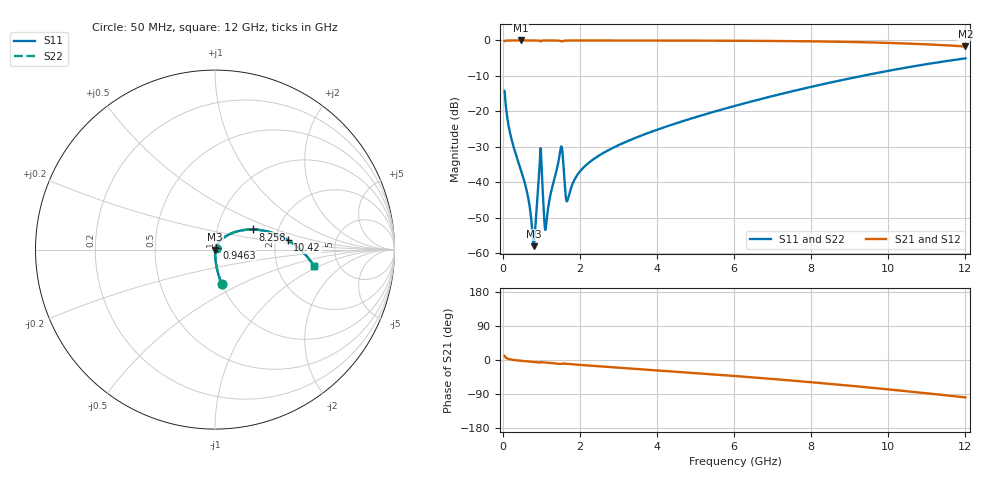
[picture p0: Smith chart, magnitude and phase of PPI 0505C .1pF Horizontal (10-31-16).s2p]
# MHz S MA R 50
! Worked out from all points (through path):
!   1601 points, 50 MHz to 12 GHz, reference 50 ohm
!   highest |S21| = -0.01 dB at 468.2 MHz (marker M1); lowest = -1.7 dB at 12 GHz (marker M2)
!   group delay of S21, straight-line fit = 22.7 ps
!   lowest |S11| = -58.1 dB at 804.3 MHz (marker M3), VSWR 1.00, Z = 50.1 - j0.0232 ohm
!   |S11| at or under -10 dB: start of sweep to 9.328 GHz
!   |S22| runs from -58.1 to -5.1 dB; largest |S21 - S12| = 0
!   S11 on the Smith chart (normalised r, x): 50 MHz: 1.00, -0.39; 946.2 MHz: 1.02, +0.02; 8.258 GHz: 1.48, +0.35; 10.42 GHz: 2.34, +0.30; 12 GHz: 3.28, -0.86
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50  0.1935 -79.1  0.9808 10.9  0.9808 10.9  0.1935 -79.1
206.8438  0.04521 -88.0  0.9984 1.3  0.9984 1.3  0.04521 -88.0
468.25  0.01514 -88.9  0.9991 -2.0  0.9991 -2.0  0.01514 -88.9
640.0312  0.006891 -85.6  0.999 -3.5  0.999 -3.5  0.006891 -85.6
804.3438  0.001246 -10.7  0.9987 -4.9  0.9987 -4.9  0.001246 -10.7
849.1562  0.00256 49.6  0.9985 -5.3  0.9985 -5.3  0.00256 49.6
946.25  0.01384 56.6  0.9936 -6.5  0.9936 -6.5  0.01384 56.6
998.5312  0.02332 -34.9  0.9796 -5.4  0.9796 -5.4  0.02332 -34.9
1080.688  0.002798 -35.1  0.9975 -6.5  0.9975 -6.5  0.002798 -35.1
1125.5  0.002428 31.0  0.998 -6.9  0.998 -6.9  0.002428 31.0
1498.938  0.02871 42.0  0.9821 -10.4  0.9821 -10.4  0.02871 42.0
1543.75  0.02857 -2.2  0.9716 -9.6  0.9716 -9.6  0.02857 -2.2
1633.375  0.006431 -7.9  0.9935 -9.9  0.9935 -9.9  0.006431 -7.9
1678.188  0.005439 29.2  0.9957 -10.4  0.9957 -10.4  0.005439 29.2
2044.156  0.01501 69.4  0.9978 -13.3  0.9978 -13.3  0.01501 69.4
4038.312  0.05569 60.3  0.9959 -27.4  0.9959 -27.4  0.05569 60.3
6025  0.1192 46.3  0.9895 -42.2  0.9895 -42.2  0.1192 46.3
8019.156  0.2224 30.2  0.9706 -58.8  0.9706 -58.8  0.2224 30.2
8258.156  0.238 28.1  0.9668 -60.9  0.9668 -60.9  0.238 28.1
10013.31  0.3733 11.6  0.9221 -77.7  0.9221 -77.7  0.3733 11.6
10416.62  0.4091 7.5  0.9066 -81.8  0.9066 -81.8  0.4091 7.5
12000  0.5586 -9.3  0.8225 -98.7  0.8225 -98.7  0.5586 -9.3
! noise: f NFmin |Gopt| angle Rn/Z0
50  0.000392  0.8724  0.4103  0.0006624
1372  0.006011  0.7835  8.323  0.005673
2701  0.006984  0.6626  16.19  0.003886
4031  0.009285  0.6354  23.8  0.004601
5360  0.01161  0.6258  31.09  0.005415
6682  0.014  0.6264  37.98  0.006311
8012  0.01653  0.6346  44.53  0.007354
9341  0.0193  0.649  50.69  0.008611
1.067e+04  0.02239  0.6683  56.49  0.01018
1.2e+04  0.02593  0.6917  61.98  0.01218
